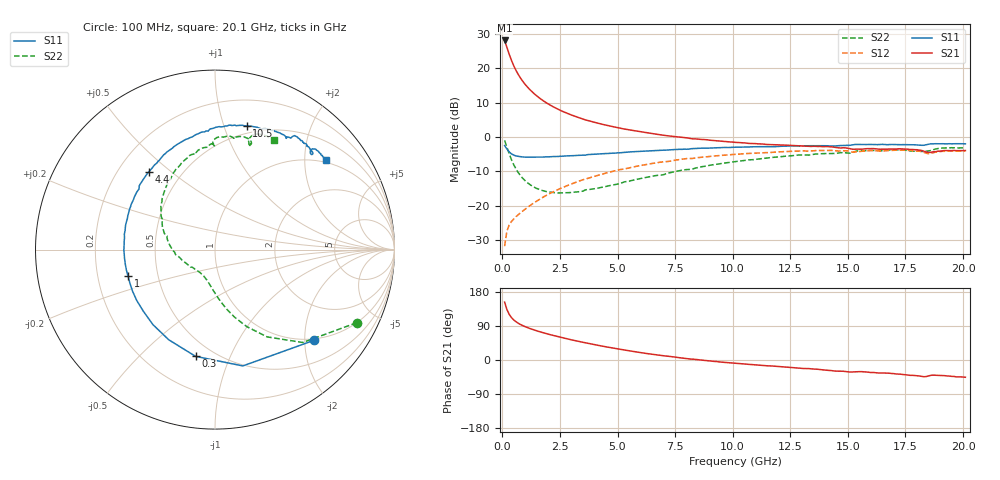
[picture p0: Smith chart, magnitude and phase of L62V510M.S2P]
!  Infineon Technologies AG
! BFR380L3 , PF131585-7, No.6, Th 09.10.01, soldered on pcb-board, measured with PP GSG850
!  Vce=2.5 V,  Ic=10.0 mA
! Common Emitter S-Parameters:  15. November 2001
#  GHz  S  MA  R  50
! f  S11  S21  S12  S22
! GHz  Mag  Ang  Mag  Ang  Mag  Ang  Mag  Ang
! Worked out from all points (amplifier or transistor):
!   201 points, 100 MHz to 20.1 GHz, reference 50 ohm
!   highest |S21| = 28.1 dB at 100 MHz (marker M1)
!   |S21| within 3 dB of that: start of sweep to 249.5 MHz
!   unconditionally stable (mu >= 1): 1.821 GHz to 4.623 GHz
!   at 3.4 GHz: K = 1.03, MAG = 8.0 dB, |S12| = -12.7 dB
!   at 10.1 GHz: K = 0.95, MSG = 1.8 dB, |S12| = -5.1 dB
!   at 20.1 GHz: K = 0.99, MSG = 0.1 dB, |S12| = -4.1 dB
!   S11 on the Smith chart (normalised r, x): 100 MHz: 0.96, -2.20; 300 MHz: 0.40, -0.75; 1 GHz: 0.33, -0.13; 4.4 GHz: 0.33, +0.42; 10.5 GHz: 0.43, +1.20; 20.1 GHz: 0.95, +2.53
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0.1  0.747 -42.7  25.42 152.7  0.02557 70.0  0.8888 -27.3
0.2  0.6664 -76.5  20.21 133.1  0.04251 57.4  0.712 -46.6
0.3  0.6045 -100.3  15.99 120.5  0.05204 51.5  0.5665 -59.1
0.4  0.5646 -117.2  12.98 111.8  0.05867 49.0  0.4633 -67.7
0.5  0.5425 -129.6  10.81 105.5  0.06387 48.5  0.3909 -73.9
0.6  0.5266 -139.3  9.23 100.7  0.06914 48.9  0.3388 -78.8
0.7  0.52 -147.0  8.043 96.7  0.07377 49.6  0.2996 -82.8
0.8  0.5147 -153.1  7.111 93.3  0.07884 50.6  0.2699 -86.3
1  0.5068 -163.0  5.782 87.7  0.08901 52.4  0.2284 -92.2
1.2  0.5062 -170.7  4.867 83.0  0.09985 53.9  0.2018 -97.4
1.4  0.5062 -177.0  4.208 78.9  0.1109 55.2  0.1836 -102.2
1.6  0.507 177.5  3.709 75.0  0.1225 56.0  0.1717 -106.7
1.9  0.5123 170.3  3.161 69.8  0.1401 56.5  0.1602 -113.0
2.6  0.523 156.9  2.366 58.9  0.1818 56.1  0.1531 -127.4
3.5  0.5414 142.4  1.819 46.6  0.2373 53.0  0.1622 -142.9
4.4  0.5696 130.2  1.509 36.0  0.2913 48.8  0.1862 -159.6
6.8  0.6356 103.7  1.08 12.7  0.4251 33.9  0.2769 165.3
10.1  0.7073 78.3  0.833 -8.5  0.5564 12.4  0.4362 129.8
10.5  0.711 75.6  0.818 -10.6  0.5687 9.7  0.4537 125.9
13.5  0.7429 60.4  0.7294 -23.8  0.6269 -8.8  0.5559 100.4
16.8  0.7736 47.8  0.6675 -34.9  0.6322 -25.0  0.6427 78.3
20.1  0.7929 38.8  0.6327 -45.6  0.6244 -38.8  0.6963 61.7
